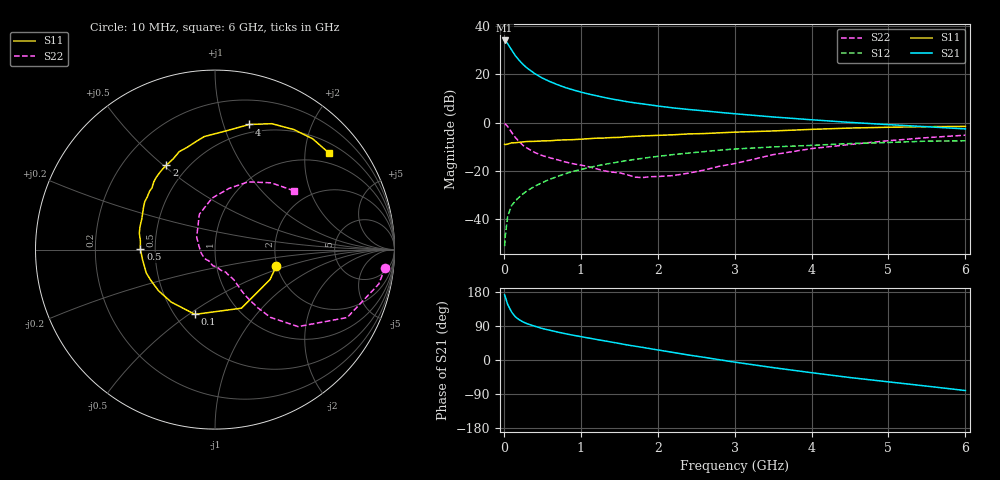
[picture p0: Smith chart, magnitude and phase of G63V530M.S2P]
! SIEMENS Small Signal Semiconductors
! BFG193
! Si NPN RF Bipolar Junction Transistor in SOT223
! VCE = 3.5 V  IC = 30 mA
! Common Emitter S-Parameters:  August  1996
# GHz  S  MA  R  50
!  f  S11  S21  S12  S22
! GHz  MAG  ANG  MAG  ANG  MAG  ANG  MAG  ANG
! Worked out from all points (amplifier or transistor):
!   36 points, 10 MHz to 6 GHz, reference 50 ohm
!   highest |S21| = 34.1 dB at 10 MHz (marker M1)
!   |S21| within 3 dB of that: start of sweep to 82.39 MHz
!   unconditionally stable (mu >= 1): 544.9 MHz to 2.421 GHz
!   at 250 MHz: K = 0.84, MSG = 26.9 dB, |S12| = -29.6 dB
!   at 1.4 GHz: K = 1.04, MAG = 12.1 dB, |S12| = -16.9 dB
!   at 6 GHz: K = 0.89, MSG = 2.5 dB, |S12| = -7.6 dB
!   S11 on the Smith chart (normalised r, x): 10 MHz: 1.98, -0.42; 100 MHz: 0.63, -0.53; 500 MHz: 0.41, +0.00; 2 GHz: 0.38, +0.51; 4 GHz: 0.42, +1.22; 6 GHz: 0.73, +2.54
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0.01  0.3542 -15.0  50.92 172.2  0.0027 85.9  0.9542 -6.0
0.02  0.349 -28.6  49.44 165.8  0.0046 83.2  0.9321 -11.9
0.05  0.3582 -65.7  43.48 146.6  0.0113 70.5  0.828 -27.2
0.1  0.3778 -107.2  32.56 126.9  0.0188 64.6  0.6311 -42.8
0.15  0.3808 -129.9  24.55 113.9  0.0236 61.7  0.4878 -50.7
0.2  0.3893 -143.9  19.64 106.3  0.0283 63.2  0.4011 -53.7
0.25  0.3964 -154.2  16.12 100.3  0.0332 62.8  0.3352 -55.6
0.3  0.4045 -161.3  13.7 96.0  0.038 64.5  0.2968 -56.8
0.4  0.4077 -172.0  10.47 89.3  0.0473 65.0  0.2398 -57.5
0.5  0.4158 179.5  8.433 83.1  0.0566 64.8  0.2061 -57.7
0.6  0.4188 173.2  7.096 78.4  0.0666 64.4  0.1857 -58.8
0.8  0.4372 162.8  5.343 69.4  0.0865 61.8  0.1516 -63.1
1.1  0.4621 149.6  3.929 58.1  0.1154 57.2  0.1212 -73.6
1.6  0.5085 132.1  2.721 39.9  0.1624 47.2  0.0828 -103.9
2  0.5425 119.9  2.212 26.6  0.1981 38.4  0.0756 -147.6
2.2  0.5572 114.6  2.021 20.0  0.2162 34.0  0.0792 -164.7
2.8  0.6118 99.8  1.633 0.8  0.2669 20.3  0.1235 145.8
3.5  0.6695 83.5  1.309 -20.1  0.312 3.2  0.2153 113.9
4  0.7227 74.7  1.144 -33.5  0.3361 -6.6  0.2879 93.1
4.5  0.7697 65.7  1.009 -46.3  0.3664 -16.7  0.3506 76.9
5.5  0.823 48.6  0.82 -69.0  0.4118 -40.1  0.4864 49.9
6  0.8322 40.3  0.739 -80.6  0.4175 -53.5  0.547 36.9
